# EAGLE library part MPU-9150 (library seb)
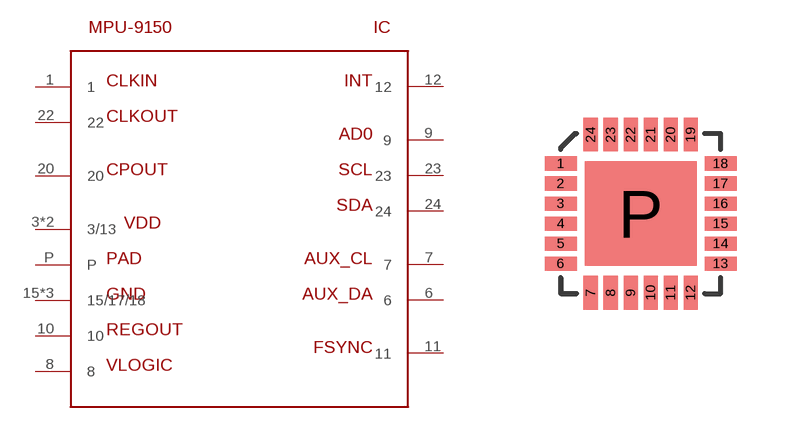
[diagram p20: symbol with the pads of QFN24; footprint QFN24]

Designator prefix IC

## MPU-9150  [QFN24]
1  1
3  3/13
6  6
7  7
8  8
9  9
10  10
11  11
12  12
13  3/13
15  15/17/18
17  15/17/18
18  15/17/18
20  20
22  22
23  23
24  24
P  P

## Footprint QFN24 (pad centres in mm)
smd 0.8 x 0.35: 1 -2,1.25; 2 -2,0.75; 3 -2,0.25; 4 -2,-0.25; 5 -2,-0.75; 6 -2,-1.25; 13 2,-1.25; 14 2,-0.75; 15 2,-0.25; 16 2,0.25; 17 2,0.75; 18 2,1.25
smd 0.35 x 0.85: 7 -1.25,-1.975; 8 -0.75,-1.975; 9 -0.25,-1.975; 10 0.25,-1.975; 11 0.75,-1.975; 12 1.25,-1.975; 19 1.25,1.975; 20 0.75,1.975; 21 0.25,1.975; 22 -0.25,1.975; 23 -0.75,1.975; 24 -1.25,1.975
smd 2.8 x 2.6: P 0,0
